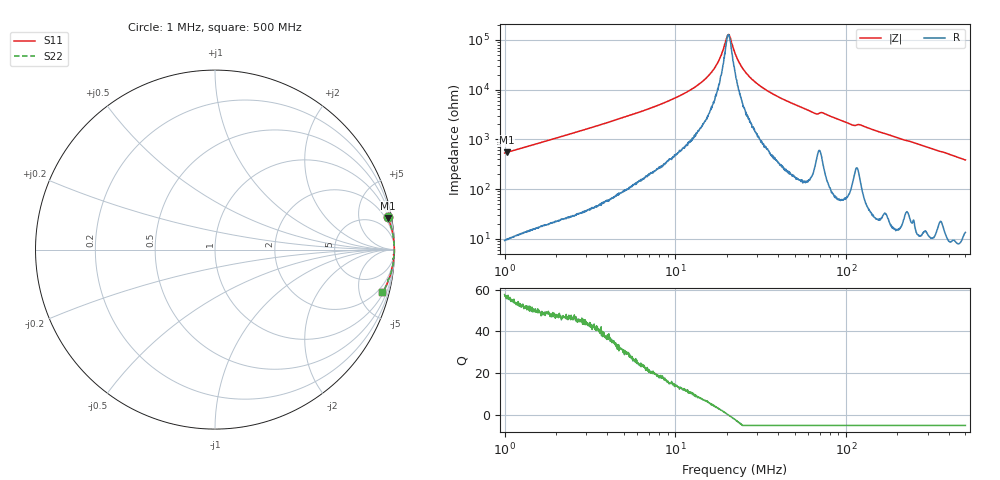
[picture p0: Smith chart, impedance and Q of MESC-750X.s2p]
!s-Parameter Generated by FASTRON Sdn. Bhd.
!FASTRON P/N : MESC-750X
!Keysight Technologies,E4991B,MY54100416,A.01.15
!Date: Fri Mar 27 10:09:13 2026
!Version  : Rev00 Fri Mar 27 10:09:13 2026
!Data & Calibration Information:
!PortZ  Port1:50+j0  Port2:50+j0
!When reading, reference impedance value at option line is always used.
! Remarks : This data is being provided solely for informational purposes.
!Freq	S11	S21	S12	S22
# Hz S dB R 50
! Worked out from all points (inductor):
!   1601 points, 1 MHz to 500 MHz, reference 50 ohm
!   read as one part in series: L = 84.1 uH near 1.032 MHz
!   highest Q = 56.3 at 1.032 MHz (marker M1), where L = 84.5 uH
!   self-resonance near 20.37 MHz
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1000000  -0.18 10.6  -14.68 -78.4  -14.68 -78.4  -0.18 10.6
1031561  -0.17 10.3  -14.94 -78.7  -14.94 -78.7  -0.17 10.3
2820919  -0.03 3.8  -23.59 -84.9  -23.59 -84.9  -0.03 3.8
7957584  -0.01 1.2  -33.80 -85.8  -33.80 -85.8  -0.01 1.2
1.18721e7  -0.01 0.6  -39.35 -84.0  -39.35 -84.0  -0.01 0.6
1.510471e7  -0.01 0.3  -44.56 -81.3  -44.56 -81.3  -0.01 0.3
1.764358e7  -0.01 0.2  -50.63 -72.9  -50.63 -72.9  -0.01 0.2
1.862957e7  -0.01 0.1  -54.07 -66.0  -54.07 -66.0  -0.01 0.1
1.99012e7  -0.01 0.0  -60.56 -33.0  -60.56 -33.0  -0.01 0.0
2.037044e7  -0.01 0.0  -62.11 -3.5  -62.11 -3.5  -0.01 0.0
2.101335e7  -0.01 -0.0  -60.89 32.7  -60.89 32.7  -0.01 -0.0
2.236068e7  -0.01 -0.1  -54.80 65.1  -54.80 65.1  -0.01 -0.1
2.370216e7  -0.01 -0.2  -50.81 74.5  -50.81 74.5  -0.01 -0.2
2.541858e7  -0.01 -0.2  -47.59 79.6  -47.59 79.6  -0.01 -0.2
3.074732e7  -0.01 -0.5  -41.97 84.3  -41.97 84.3  -0.01 -0.5
4.019762e7  -0.01 -0.8  -37.06 86.5  -37.06 86.5  -0.01 -0.8
6.307767e7  -0.02 -1.6  -31.03 85.4  -31.03 85.4  -0.02 -1.6
7.310989e7  -0.03 -1.7  -30.70 82.8  -30.70 82.8  -0.03 -1.7
1.082302e8  -0.04 -2.9  -25.90 83.7  -25.90 83.7  -0.04 -2.9
1.211344e8  -0.04 -2.9  -25.88 82.9  -25.88 82.9  -0.04 -2.9
1.77937e8  -0.04 -4.6  -21.89 84.3  -21.89 84.3  -0.04 -4.6
5e8  -0.36 -14.4  -12.08 73.6  -12.08 73.6  -0.36 -14.4
